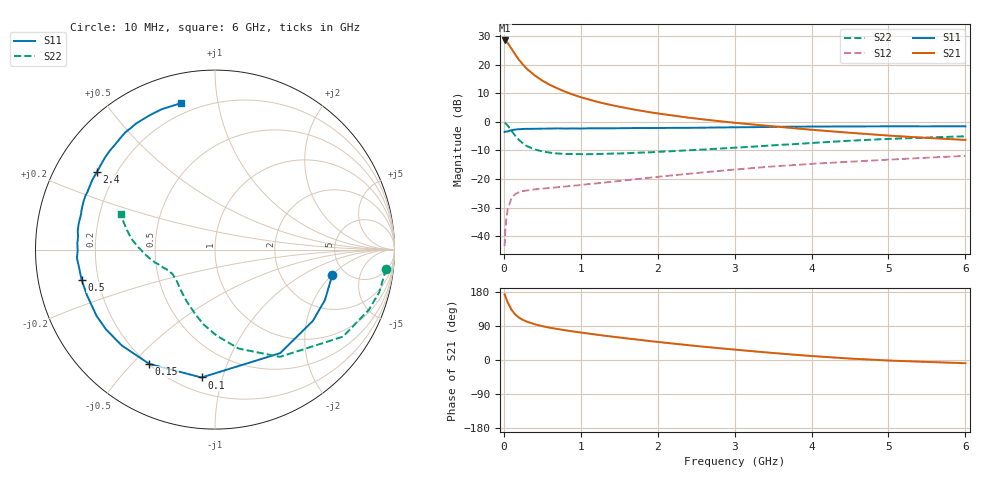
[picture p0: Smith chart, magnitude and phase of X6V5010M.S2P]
! SIEMENS Small Signal Semiconductors
! BFP193W
! Si NPN RF Bipolar Junction Transistor in SOT343
! VCE = 0.5 V  IC = 10 mA
! Common Emitter S-Parameters:  April 1994
# GHz  S  MA  R  50
!  f  S11  S21  S12  S22
! GHz  MAG  ANG  MAG  ANG  MAG  ANG  MAG  ANG
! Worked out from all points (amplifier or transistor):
!   40 points, 10 MHz to 6 GHz, reference 50 ohm
!   highest |S21| = 28.5 dB at 10 MHz (marker M1)
!   |S21| within 3 dB of that: start of sweep to 102.8 MHz
!   unconditionally stable (mu >= 1): 1.132 GHz to end of sweep
!   at 200 MHz: K = 0.24, MSG = 23.1 dB, |S12| = -24.6 dB
!   at 1.5 GHz: K = 1.15, MAG = 10.7 dB, |S12| = -20.7 dB
!   at 6 GHz: K = 1.09, MAG = 1.0 dB, |S12| = -11.9 dB
!   S11 on the Smith chart (normalised r, x): 10 MHz: 3.92, -2.04; 100 MHz: 0.29, -0.86; 150 MHz: 0.20, -0.56; 500 MHz: 0.14, -0.11; 2.4 GHz: 0.13, +0.29; 6 GHz: 0.14, +0.79
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0.01  0.6685 -12.4  26.58 173.3  0.0067 83.9  0.9593 -6.4
0.02  0.674 -24.7  26.32 168.2  0.0133 79.1  0.9457 -14.5
0.03  0.6746 -36.1  25.84 162.6  0.019 73.4  0.9209 -21.3
0.05  0.6816 -57.8  24.06 152.1  0.0296 64.3  0.8626 -34.2
0.1  0.7165 -96.0  19.07 132.5  0.0464 47.7  0.6986 -58.8
0.15  0.7349 -119.9  14.96 119.6  0.0549 37.9  0.5669 -76.6
0.2  0.7451 -134.2  12.02 111.5  0.0592 32.5  0.4777 -89.2
0.25  0.7526 -143.9  10.01 105.6  0.0617 29.1  0.4208 -98.9
0.3  0.7563 -150.9  8.48 101.2  0.0631 27.3  0.3771 -106.7
0.4  0.7573 -160.5  6.516 94.4  0.066 25.7  0.33 -118.3
0.5  0.7622 -167.3  5.283 89.3  0.068 25.8  0.3042 -126.6
0.6  0.7638 -172.3  4.432 85.1  0.07 26.1  0.2895 -133.0
0.8  0.765 -179.7  3.36 78.4  0.0741 28.5  0.2752 -141.3
1.1  0.7717 172.3  2.479 69.8  0.0816 31.8  0.2725 -148.6
1.3  0.7723 167.6  2.107 64.4  0.0866 34.1  0.276 -151.7
1.6  0.7781 161.3  1.736 56.9  0.0957 36.6  0.2828 -155.4
2.2  0.7863 150.2  1.291 43.4  0.1164 39.4  0.3082 -161.7
2.4  0.7872 146.8  1.186 39.1  0.1235 39.6  0.3186 -163.5
3.2  0.8078 133.6  0.911 23.8  0.1542 38.6  0.3669 -172.3
4.5  0.8323 115.9  0.645 3.8  0.2012 32.8  0.469 172.7
5.5  0.8353 107.0  0.525 -5.1  0.2363 27.7  0.5331 163.1
6  0.8377 102.9  0.484 -8.4  0.2543 25.3  0.5598 159.3
